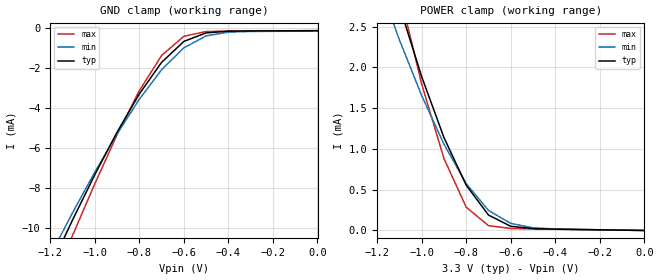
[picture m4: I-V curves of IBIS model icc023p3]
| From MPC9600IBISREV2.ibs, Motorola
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|This is a Model of an Input with a 25,000 ohm Pull_up at 3.3V
[Model]   icc023p3
Model_type   Input
Polarity   Non-Inverting
Vmeas=1.5
Vinl=0.8
Vinh=2.0
|Variable   typ   min   max
C_comp   5p   5p   5p
[Temperature Range]   27.00   100.00   -45.00
[Power Clamp Reference]   3.30V   3.00V   3.60V
[Gnd Clamp Reference]   0.000V   0.000V   0.000V
[Voltage Range]   3.30V   3.00V   3.60V
[Pulldown Reference]   0.000V   0.000V   0.000V
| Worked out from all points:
|   GND clamp passes 1 mA (typ) near -0.63 V on its own axis
|   POWER clamp passes 1 mA (typ) near -0.88 V on its own axis
[GND_clamp]
| voltage   I(typ)   I(min)   I(max)
-3.3V     -65.56mA   -61.83mA   -70.36mA
-1.2V     -11.94mA   -11.35mA   -13.02mA
-1.1V     -9.583mA   -9.224mA   -10.36mA
-1V       -7.318mA   -7.188mA   -7.771mA
-900mV    -5.193mA   -5.279mA   -5.323mA
-800mV    -3.28mA    -3.546mA   -3.115mA
-700mV    -1.702mA   -2.069mA   -1.359mA
-600mV    -655uA     -975.9uA   -396.7uA
-500mV    -229.7uA   -377.6uA   -163.2uA
-400mV    -143.9uA   -192.2uA   -135.8uA
1.97fV    -118.8uA   -142.6uA   -118.8uA
[POWER_clamp]
| voltage   I(typ)  I(min)  I(max)
-3.3V     32.89mA    26.85mA    40.63mA
-1.2V     3.727mA    3.095mA    4.229mA
-1.1V     2.756mA    2.338mA    2.93mA
-1V       1.886mA    1.654mA    1.795mA
-900mV    1.14mA     1.058mA    882.5uA
-800mV    554.8uA    575uA      285.5uA
-700mV    189.3uA    245.4uA    59.28uA
-600mV    51.31uA    86.95uA    24.32uA
-500mV    23.2uA     32.54uA    18.63uA
-400mV    16.45uA    18.02uA    14.85uA
0V        148.9pA    557.5pA    4.024pA
